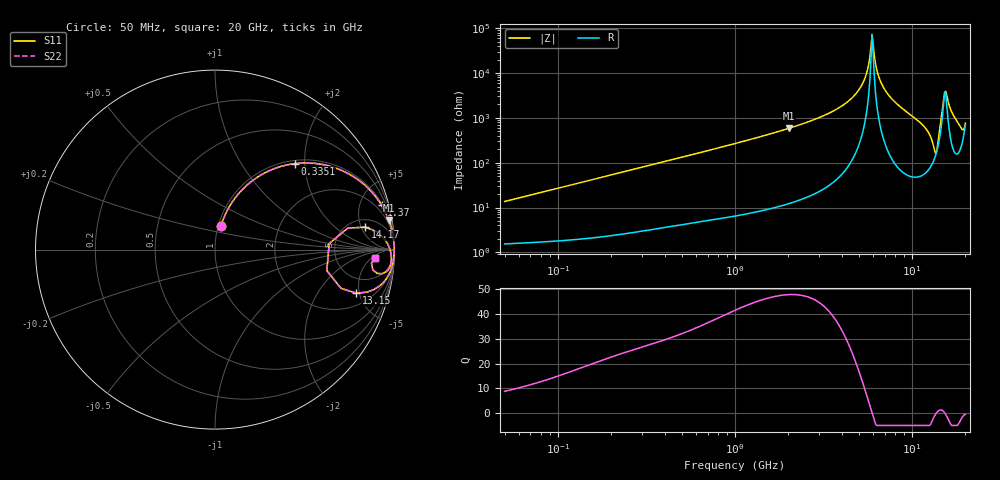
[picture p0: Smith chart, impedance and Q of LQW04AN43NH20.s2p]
!Murata Part Number: LQW04AN43NH20
!These Parameters are Measured in Series Mode Connection
!  o--[Z]--o
!Port1  Port2
!  o-------o
!Freq. Start=50[MHz] Stop=20[GHz], 401[Steps]
# Hz S RI R 50
!Freq.(Hz) S11(Real) S11(Imag) S21(Real) S21(Imag) S12(Real) S12(Imag) S22(Real) S22(Imag)
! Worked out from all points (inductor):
!   401 points, 50 MHz to 20 GHz, reference 50 ohm
!   read as one part in series: L = 42.9 nH near 51.52 MHz
!   highest Q = 47.9 at 2.022 GHz (marker M1), where L = 46.2 nH
!   self-resonance near 5.944 GHz
!   S11 on the Smith chart (normalised r, x): 50 MHz: 1.03, +0.27; 335.1 MHz: 1.06, +1.77; 1.37 GHz: 1.16, +7.47; 13.15 GHz: 3.08, -4.67; 14.17 GHz: 6.73, +5.98; 20 GHz: 15, -7
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5e7  0.0323 0.1289  0.9677 -0.1289  0.9677 -0.1289  0.0323 0.1289
1.364002e8  0.1306 0.3109  0.8694 -0.3109  0.8694 -0.3109  0.1306 0.3109
3.350611e8  0.4429 0.4791  0.5571 -0.4791  0.5571 -0.4791  0.4429 0.4791
3.721004e8  0.4928 0.4829  0.5072 -0.4829  0.5072 -0.4829  0.4928 0.4829
1e9  0.8712 0.3231  0.1288 -0.3231  0.1288 -0.3231  0.8712 0.3231
1.369645e9  0.9285 0.2469  0.0715 -0.2469  0.0715 -0.2469  0.9285 0.2469
2.021818e9  0.9685 0.1644  0.0315 -0.1644  0.0315 -0.1644  0.9685 0.1644
2.728004e9  0.9849 0.1116  0.0151 -0.1116  0.0151 -0.1116  0.9849 0.1116
3.850025e9  0.9947 0.0596  0.00525 -0.0596  0.00525 -0.0596  0.9947 0.0596
4.81993e9  0.9978 0.0287  0.00224 -0.0287  0.00224 -0.0287  0.9978 0.0287
5.433528e9  0.9985 0.0125  0.00152 -0.0125  0.00152 -0.0125  0.9985 0.0125
5.944466e9  0.9986 0.000195  0.00136 -0.000195  0.00136 -0.000195  0.9986 0.000195
6.601595e9  0.9984 -0.0145  0.00164 0.0145  0.00164 0.0145  0.9984 -0.0145
7.442007e9  0.9973 -0.0324  0.00268 0.0324  0.00268 0.0324  0.9973 -0.0324
1.183995e10  0.9594 -0.1554  0.0406 0.1554  0.0406 0.1554  0.9594 -0.1554
1.314879e10  0.7878 -0.2428  0.2122 0.2428  0.2122 0.2428  0.7878 -0.2428
1.375312e10  0.6361 0.0332  0.3639 -0.0332  0.3639 -0.0332  0.6361 0.0332
1.417136e10  0.8382 0.1252  0.1618 -0.1252  0.1618 -0.1252  0.8382 0.1252
1.504638e10  0.9669 0.0217  0.0331 -0.0217  0.0331 -0.0217  0.9669 0.0217
1.550395e10  0.9784 -0.0127  0.0216 0.0127  0.0216 0.0127  0.9784 -0.0127
1.828096e10  0.9554 -0.1219  0.0446 0.1219  0.0446 0.1219  0.9554 -0.1219
2e10  0.8923 -0.0454  0.1077 0.0454  0.1077 0.0454  0.8923 -0.0454
